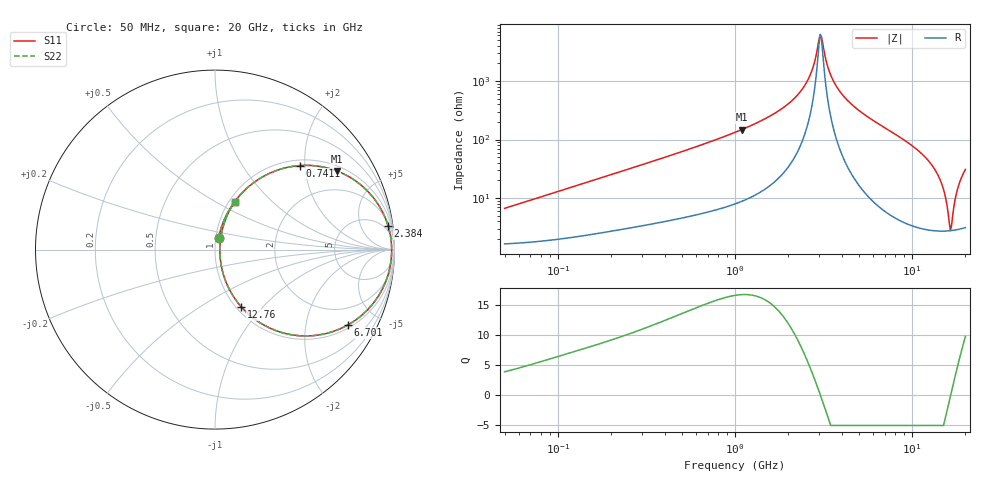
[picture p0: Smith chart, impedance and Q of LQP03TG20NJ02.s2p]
!Murata Part Number: LQP03TG20NJ02
!These Parameters are Measured in Series Mode Connection
!  o--[Z]--o
!Port1  Port2
!  o-------o
!Freq. Start=50[MHz] Stop=20[GHz], 401[Steps]
# Hz S RI R 50
!Freq.(Hz) S11(Real) S11(Imag) S21(Real) S21(Imag) S12(Real) S12(Imag) S22(Real) S22(Imag)
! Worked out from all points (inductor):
!   401 points, 50 MHz to 20 GHz, reference 50 ohm
!   read as one part in series: L = 20.6 nH near 51.52 MHz
!   highest Q = 16.8 at 1.094 GHz (marker M1), where L = 21.6 nH
!   self-resonance near 3.03 GHz
!   S11 on the Smith chart (normalised r, x): 50 MHz: 1.03, +0.13; 741.1 MHz: 1.12, +1.88; 2.384 GHz: 3, +14; 6.701 GHz: 1.13, -3.46; 12.76 GHz: 1.06, -0.77; 20 GHz: 1.06, +0.62
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5e7  0.0202 0.0625  0.9798 -0.0625  0.9798 -0.0625  0.0202 0.0625
1.364002e8  0.0493 0.161  0.9507 -0.161  0.9507 -0.161  0.0493 0.161
3.721004e8  0.195 0.357  0.805 -0.357  0.805 -0.357  0.195 0.357
7.411344e8  0.4713 0.4681  0.5287 -0.4681  0.5287 -0.4681  0.4713 0.4681
1e9  0.6304 0.4536  0.3696 -0.4536  0.3696 -0.4536  0.6304 0.4536
1.094034e9  0.6779 0.4384  0.3221 -0.4384  0.3221 -0.4384  0.6779 0.4384
1.766834e9  0.89 0.2793  0.11 -0.2793  0.11 -0.2793  0.89 0.2793
2.383959e9  0.9643 0.1324  0.0357 -0.1324  0.0357 -0.1324  0.9643 0.1324
2.728004e9  0.98 0.06  0.02 -0.06  0.02 -0.06  0.98 0.06
2.98453e9  0.9842 0.0103  0.0158 -0.0103  0.0158 -0.0103  0.9842 0.0103
3.075291e9  0.9844 -0.00649  0.0156 0.00649  0.0156 0.00649  0.9844 -0.00649
3.415248e9  0.9804 -0.0656  0.0196 0.0656  0.0196 0.0656  0.9804 -0.0656
3.908127e9  0.9638 -0.1421  0.0362 0.1421  0.0362 0.1421  0.9638 -0.1421
6.701223e9  0.7418 -0.419  0.2582 0.419  0.2582 0.419  0.7418 -0.419
7.442007e9  0.6638 -0.4543  0.3362 0.4543  0.3362 0.4543  0.6638 -0.4543
9.892087e9  0.3979 -0.4688  0.6021 0.4688  0.6021 0.4688  0.3979 -0.4688
1.276073e10  0.1473 -0.3199  0.8527 0.3199  0.8527 0.3199  0.1473 -0.3199
1.482269e10  0.0498 -0.1485  0.9502 0.1485  0.9502 0.1485  0.0498 -0.1485
1.646126e10  0.027 -0.00307  0.973 0.00307  0.973 0.00307  0.027 -0.00307
1.696185e10  0.029 0.0401  0.971 -0.0401  0.971 -0.0401  0.029 0.0401
1.828096e10  0.0511 0.147  0.9489 -0.147  0.9489 -0.147  0.0511 0.147
2e10  0.1097 0.2657  0.8903 -0.2657  0.8903 -0.2657  0.1097 0.2657
